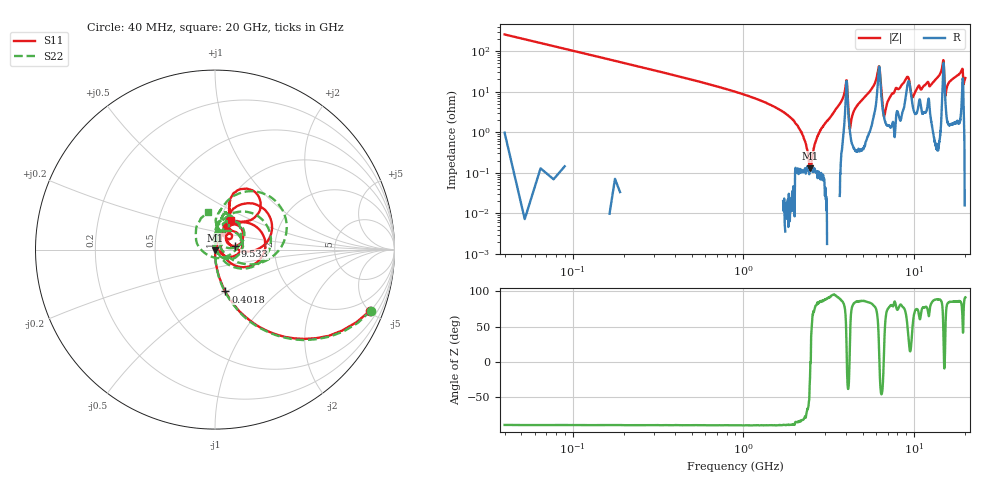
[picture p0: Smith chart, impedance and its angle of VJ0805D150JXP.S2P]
! VJ0805D150JXP
! DATE 10/29/2021  12:12
! CAPACITORS MOUNTED IN SERIES ON 25 MIL THICK MICROSTRIP SUBSTRATE
# GHz  S  MA  R  50.00
!  FREQ  S11M  S11A  S21M  S21A  S12M  S12A  S22M  S22A
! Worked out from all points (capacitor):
!   1601 points, 40 MHz to 20 GHz, reference 50 ohm
!   read as one part in series: C = 15.5 pF near 139.8 MHz
!   lowest |Z| = 130 mohm at 2.473 GHz (marker M1)
!   series resonance near 2.486 GHz, so ESL is about 260 pH
!   S11 on the Smith chart (normalised r, x): 40 MHz: 1.02, -5.06; 401.8 MHz: 1.00, -0.49; 9.533 GHz: 1.25, +0.05; 20 GHz: 1.13, +0.38
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0.04  0.9285 -21.6  0.363 68.3  0.3653 68.3  0.9333 -21.4
0.401775  0.2399 -76.1  0.9698 13.9  0.9701 14.0  0.2438 -76.3
1.9362  0.02371 -87.5  0.9991 1.1  0.999 1.0  0.02427 -89.9
2.472625  0.004111 -53.8  0.9978 -0.2  0.999 -0.2  0.004033 -96.4
2.622325  0.003101 12.8  0.998 -0.5  0.9995 -0.6  0.0008236 130.9
3.370825  0.02057 83.1  1.002 -2.0  1.003 -2.1  0.02722 105.1
3.994575  0.1413 48.4  0.9078 -7.1  0.9086 -7.2  0.1432 44.7
4.25655  0.01648 25.9  0.9911 -1.0  0.9919 -1.1  0.00917 96.2
4.543475  0.03445 68.8  0.9955 -2.5  0.9953 -2.6  0.03604 95.8
6.215125  0.2807 16.1  0.7343 -9.7  0.7351 -9.8  0.3173 27.4
6.70165  0.03459 7.1  0.9783 -1.1  0.9783 -1.2  0.009433 21.7
7.7745  0.1056 70.1  0.984 -7.0  0.9842 -7.1  0.1065 80.4
9.14675  0.187 37.1  0.864 -9.7  0.8649 -9.8  0.1993 44.1
9.533475  0.1143 10.3  0.8997 -2.1  0.9006 -2.3  0.08169 5.8
10.02  0.08411 44.3  0.9659 -4.9  0.9653 -5.1  0.06773 81.1
13.35083  0.181 66.0  0.9772 -12.0  0.9776 -12.2  0.1795 87.9
14.83535  0.3559 31.4  0.687 -19.7  0.6873 -19.8  0.4338 27.0
15.27197  0.08499 24.5  0.9365 -3.9  0.9369 -4.1  0.03476 50.8
16.68165  0.1607 68.6  0.9662 -12.4  0.9672 -12.7  0.1796 77.9
18.9521  0.2978 73.2  0.9094 -20.3  0.9108 -20.6  0.1988 53.6
19.36378  0.3587 44.9  0.7873 -9.7  0.7876 -9.8  0.04398 -116.2
20  0.1874 61.0  0.9707 -13.6  0.9715 -13.9  0.2126 101.1
